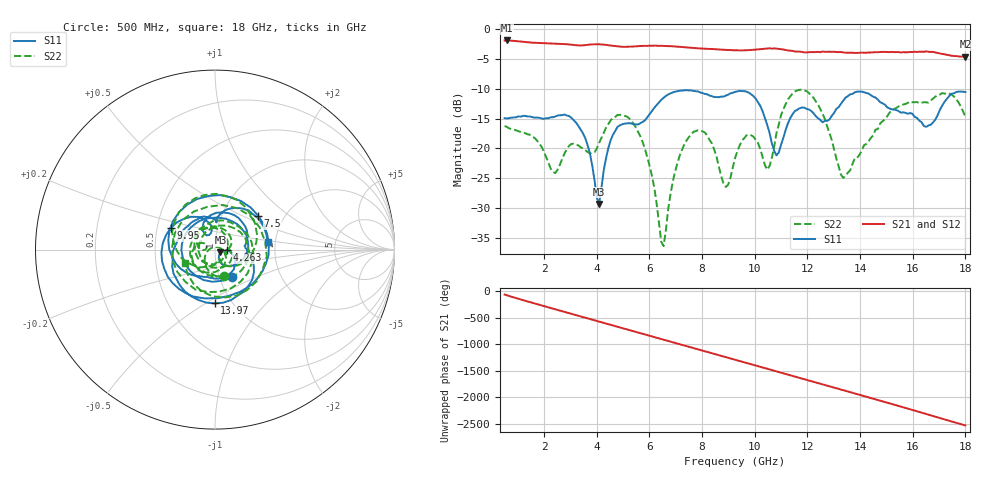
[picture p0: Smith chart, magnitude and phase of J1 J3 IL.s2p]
!Agilent Technologies,N5230A,MY45001360,A.07.50.67
!Agilent N5230A: A.07.50.67
!Date: Tuesday, April 16, 2024 16:23:51
!Correction: S11(Full 2 Port(1,2))
!S21(Full 2 Port(1,2))
!S12(Full 2 Port(1,2))
!S22(Full 2 Port(1,2))
!S2P File: Measurements: S11, S21, S12, S22:
# Hz S  dB  R 50
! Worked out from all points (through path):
!   201 points, 500 MHz to 18 GHz, reference 50 ohm
!   highest |S21| = -1.92 dB at 587.5 MHz (marker M1); lowest = -4.7 dB at 18 GHz (marker M2)
!   group delay of S21, straight-line fit = 390 ps
!   lowest |S11| = -29.3 dB at 4.088 GHz (marker M3), VSWR 1.07, Z = 53.1 - j1.66 ohm
!   |S11| at or under -10 dB: start of sweep to end of sweep
!   |S22| runs from -36.4 to -10.2 dB; largest |S21 - S12| = 0.0081
!   S11 on the Smith chart (normalised r, x): 500 MHz: 1.15, -0.36; 4.263 GHz: 1.14, -0.01; 7.5 GHz: 1.48, +0.62; 9.95 GHz: 0.59, +0.15; 13.97 GHz: 0.83, -0.55; 18 GHz: 1.82, +0.18
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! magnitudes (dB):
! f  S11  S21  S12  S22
! 500 MHz  -14.9  -1.9  -1.9  -16.2
! 587.5 MHz  -15.0  -1.9  -1.9  -16.4
! 2.425 GHz  -14.6  -2.5  -2.5  -24.1
! 3.475 GHz  -17.5  -2.7  -2.7  -20.0
! 4.088 GHz  -29.3  -2.6  -2.6  -19.1
! 4.263 GHz  -23.7  -2.6  -2.6  -17.3
! 5.4 GHz  -16.0  -2.9  -2.9  -15.9
! 6.362 GHz  -12.3  -2.8  -2.8  -32.5
! 6.537 GHz  -11.5  -2.8  -2.8  -36.4
! 7.5 GHz  -10.3  -3.1  -3.1  -18.1
! 8.2 GHz  -11.0  -3.3  -3.3  -17.9
! 8.9 GHz  -11.2  -3.5  -3.5  -26.4
! 9.25 GHz  -10.5  -3.6  -3.6  -21.6
! 9.95 GHz  -11.2  -3.5  -3.5  -18.0
! 10.47 GHz  -16.1  -3.3  -3.3  -23.6
! 10.82 GHz  -21.1  -3.3  -3.3  -17.4
! 12.22 GHz  -14.1  -3.9  -3.8  -11.5
! 13.36 GHz  -12.0  -3.9  -3.9  -24.9
! 13.97 GHz  -10.5  -4.0  -4.0  -21.1
! 15.11 GHz  -13.3  -3.9  -3.8  -14.1
! 16.51 GHz  -16.4  -3.7  -3.8  -12.3
! 18 GHz  -10.5  -4.7  -4.7  -14.7
